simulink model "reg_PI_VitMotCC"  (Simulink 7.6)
settings: Solver=ode15s  StartTime=0.0  StopTime=5  RelTol=1e-3
InitFcn:
  | clear all
  | N=300;
  | clc
  | 
  | Ti=0.0001;
  | Kp=1.2;
  | 
  | R1=1e3;
  | R2=(Kp-1)*R1;
  | 
  | C2= Ti/(R1+R2);
StopFcn:
  | close all, clc
  | load reg_vit_PI.mat
  | plot(x(1,:),x(2,:),x(1,:),x(3,:))
  | title('Consigne et vitesse de la masse (m)')
  | axis([0 5 -0.2 1.2])
  | xlabel('temps')
  | grid
libraries: fl_lib x13, nesl_utility x5, elec_lib x1

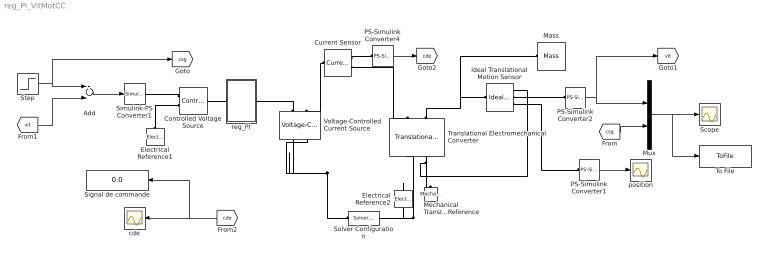
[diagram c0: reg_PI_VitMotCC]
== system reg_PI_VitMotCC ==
  Add : Sum  Inputs=+-
  Controlled Voltage Source : fl_lib/Electrical/Electrical Sources/Controlled Voltage Source  DialogController=NetworkEngine.DynNeDlgSource  SystemSampleTime=-1  i_Log=off  v_Log=off  LocalVarNames=|i|v  LocalVarDescs=|i|v  LocalVarLogging=[0 0]
  Current Sensor : fl_lib/Electrical/Electrical Sensors/Current Sensor  DialogController=NetworkEngine.DynNeDlgSource  SystemSampleTime=-1  i1_Log=off  v1_Log=off  LocalVarNames=|i1|v1  LocalVarDescs=|i1|v1  LocalVarLogging=[0 0]
  Electrical Reference1 : fl_lib/Electrical/Electrical Elements/Electrical Reference  DialogController=NetworkEngine.DynNeDlgSource  SystemSampleTime=-1  i_Log=off  LocalVarNames=|i  LocalVarDescs=|i  LocalVarLogging=[]
  Electrical Reference2 : fl_lib/Electrical/Electrical Elements/Electrical Reference  DialogController=NetworkEngine.DynNeDlgSource  SystemSampleTime=-1  i_Log=off  LocalVarNames=|i  LocalVarDescs=|i  LocalVarLogging=[]
  Ideal Translational Motion Sensor : fl_lib/Mechanical/Mechanical Sensors/Ideal Translational Motion Sensor  DialogController=NetworkEngine.DynNeDlgSource  SystemSampleTime=-1  offset=0 m  v_Log=off  f_Log=off  x_Log=off  LocalVarNames=|v|f|x  LocalVarDescs=|v|f|x  LocalVarLogging=[0 0 0]
  Mass : fl_lib/Mechanical/Translational Elements/Mass  DialogController=NetworkEngine.DynNeDlgSource  SystemSampleTime=-1  mass=0.5 kg  initial_velocity=0 m/s  f_Log=off  LocalVarNames=|f  LocalVarDescs=|f  LocalVarLogging=0
  Mechanical Translational Reference : fl_lib/Mechanical/Translational Elements/Mechanical Translational Reference  DialogController=NetworkEngine.DynNeDlgSource  SystemSampleTime=-1  f_Log=off  LocalVarNames=|f  LocalVarDescs=|f  LocalVarLogging=0
  Mux : Mux  Inputs=2
  PS-Simulink Converter1 : nesl_utility/PS-Simulink Converter  DialogController=NetworkEngine.DynNeUtilDlgSource  SystemSampleTime=-1  PhysicalDomain=network_engine_domain  LeftPortType=input  RightPortType=output  SubClassName=ps_output  Unit=1  AffineConversion=off
  PS-Simulink Converter2 : nesl_utility/PS-Simulink Converter  DialogController=NetworkEngine.DynNeUtilDlgSource  SystemSampleTime=-1  PhysicalDomain=network_engine_domain  LeftPortType=input  RightPortType=output  SubClassName=ps_output  Unit=1  AffineConversion=off
  PS-Simulink Converter4 : nesl_utility/PS-Simulink Converter  DialogController=NetworkEngine.DynNeUtilDlgSource  SystemSampleTime=-1  PhysicalDomain=network_engine_domain  LeftPortType=input  RightPortType=output  SubClassName=ps_output  Unit=1  AffineConversion=off
  Scope : Scope
  Signal de commande : Display
  Simulink-PS Converter1 : nesl_utility/Simulink-PS Converter  DialogController=NetworkEngine.DynNeUtilDlgSource  SystemSampleTime=-1  PhysicalDomain=network_engine_domain  LeftPortType=input  RightPortType=output  SubClassName=ps_input  Unit=1  AffineConversion=off  InputFilterTimeConstant=.001  UdotUserProvided=0
  Solver Configuration : nesl_utility/Solver Configuration  DialogController=NetworkEngine.DynNeUtilDlgSource  SystemSampleTime=-1  PhysicalDomain=network_engine_domain  LeftPortType=input  RightPortType=generic  SubClassName=solver  Accelerate=off  Profile=off  ResidualTolerance=1e-9  MaxNonlinIter=12  MaxModeIter=2  DoFixedCost=off  UseLocalSampling=off  DoDC=off  LinearAlgebra=Sparse  LocalSolverSampleTime=.001  LocalSolverChoice=NE_BACKWARD_EULER_ADVANCER  UseLocalSolver=off
  Step : Step  SampleTime=0
  To File : ToFile  Filename=reg_vit_PI  MatrixName=x
  Translational Electromechanical Converter : fl_lib/Electrical/Electrical Elements/Translational Electromechanical Converter  DialogController=NetworkEngine.DynNeDlgSource  SystemSampleTime=-1  K=0.1 s*V/m  i_Log=off  v_Log=off  f_Log=off  u_Log=off  LocalVarNames=|i|v|f|u  LocalVarDescs=|i|v|f|u  LocalVarLogging=[0 0 0 0]
  Voltage-Controlled Current Source : fl_lib/Electrical/Electrical Sources/Voltage-Controlled Current Source  DialogController=NetworkEngine.DynNeDlgSource  SystemSampleTime=-1  K=1 1/Ohm  i1_Log=off  v1_Log=off  i2_Log=off  v2_Log=off  LocalVarNames=|i1|v1|i2|v2  LocalVarDescs=|i1|v1|i2|v2  LocalVarLogging=[0 0 0 0]
  cde : Scope
  position : Scope
  reg_PI : Subsystem
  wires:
  Mux/1 -> Scope/1, To File/1
  PS-Simulink Converter2/1 -> Mux/1, [vit]
  PS-Simulink Converter1/1 -> position/1
  [csg] -> Mux/2
  [vit] -> Add/2
  Add/1 -> Simulink-PS Converter1/1
  Step/1 -> Add/1, [csg]
  PS-Simulink Converter4/1 -> [cde]
  [cde] -> cde/1, Signal de commande/1
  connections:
  Translational Electromechanical Converter/LConn2 -- Ideal Translational Motion Sensor/LConn1 -- Mass/LConn1
  Controlled Voltage Source/LConn1 -- reg_PI/LConn1
  Controlled Voltage Source/RConn1 -- Simulink-PS Converter1/RConn1
  Electrical Reference1/LConn1 -- Controlled Voltage Source/RConn2
  Solver Configuration/RConn1 -- Electrical Reference2/LConn1 -- Translational Electromechanical Converter/RConn1 -- Voltage-Controlled Current Source/RConn1 -- Voltage-Controlled Current Source/RConn2
  Ideal Translational Motion Sensor/RConn2 -- PS-Simulink Converter2/LConn1
  Translational Electromechanical Converter/RConn2 -- Mechanical Translational Reference/LConn1 -- Ideal Translational Motion Sensor/RConn1
  Voltage-Controlled Current Source/LConn1 -- reg_PI/RConn1
  Ideal Translational Motion Sensor/RConn3 -- PS-Simulink Converter1/LConn1
  Current Sensor/LConn1 -- Voltage-Controlled Current Source/LConn2
  Current Sensor/RConn2 -- Translational Electromechanical Converter/LConn1
  Current Sensor/RConn1 -- PS-Simulink Converter4/LConn1

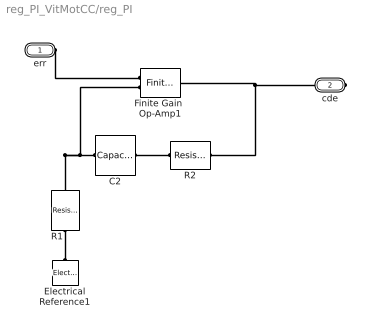
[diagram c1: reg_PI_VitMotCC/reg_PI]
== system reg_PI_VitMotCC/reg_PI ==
  C2 : fl_lib/Electrical/Electrical Elements/Capacitor  DialogController=NetworkEngine.DynNeDlgSource  SystemSampleTime=-1  c=C2 F  v0=0 V  r=1e-6 Ohm  g=0 1/Ohm  i_Log=off  v_Log=off  vc_Log=off  LocalVarNames=|i|v|vc  LocalVarDescs=|i|v|Internal variable for voltage across capacitor term  LocalVarLogging=[0 0 0]
  Electrical Reference1 : fl_lib/Electrical/Electrical Elements/Electrical Reference  DialogController=NetworkEngine.DynNeDlgSource  SystemSampleTime=-1  i_Log=off  LocalVarNames=|i  LocalVarDescs=|i  LocalVarLogging=[]
  Finite Gain  Op-Amp1 : elec_lib/Integrated Circuits/Finite Gain Op-Amp  DialogController=NetworkEngine.DynNeDlgSource  SystemSampleTime=-1  A=1000  Rin=1e+6 Ohm  Rout=100 Ohm  Vmin=-15 V  Vmax=15 V  LocalVarLogging=[]
  R1 : fl_lib/Electrical/Electrical Elements/Resistor  DialogController=NetworkEngine.DynNeDlgSource  SystemSampleTime=-1  R=R1 Ohm  i_Log=off  v_Log=off  LocalVarNames=|current|voltage|power  LocalVarDescs=|Resistor current (A)|Voltage across resistor (V)|Power (W)  LocalVarLogging=[0 0 0]
  R2 : fl_lib/Electrical/Electrical Elements/Resistor  DialogController=NetworkEngine.DynNeDlgSource  SystemSampleTime=-1  R=R2 Ohm  i_Log=off  v_Log=off  LocalVarNames=|current|voltage|power  LocalVarDescs=|Resistor current (A)|Voltage across resistor (V)|Power (W)  LocalVarLogging=[0 0 0]
  err : PMIOPort  Port=1  Side=Left
  cde : PMIOPort  Port=2  Side=Right
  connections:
  R2/RConn1 -- cde/RConn1 -- Finite Gain  Op-Amp1/RConn1
  C2/LConn1 -- Finite Gain  Op-Amp1/LConn2 -- R1/RConn1
  C2/RConn1 -- R2/LConn1
  R1/LConn1 -- Electrical Reference1/LConn1
  err/RConn1 -- Finite Gain  Op-Amp1/LConn1
